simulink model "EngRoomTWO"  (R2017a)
settings: Solver=VariableStepAuto  StartTime=0.0  StopTime=10.0  RelTol=1e-3
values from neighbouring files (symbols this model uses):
  EngDat = engine_pre()    [run_master.m]    (also in engine_pre.m = [MCR1, BSFC1, x)
undefined symbols (not defined in the file or in its folder): num

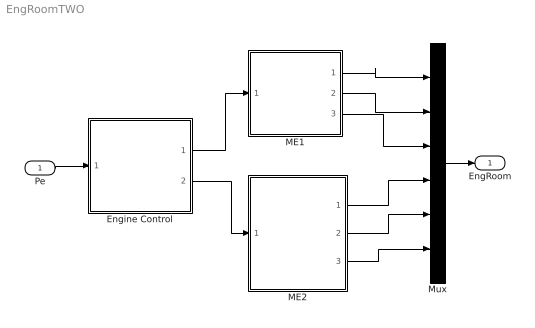
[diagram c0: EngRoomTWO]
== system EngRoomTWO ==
  Pe : Inport
  Engine Control : MATLAB Function  TreatAsAtomicUnit=on
  ME1 : MATLAB Function  TreatAsAtomicUnit=on
  ME2 : MATLAB Function  TreatAsAtomicUnit=on
  Mux : Mux  Inputs=6
  EngRoom : Outport
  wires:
  Pe/1 -> Engine Control/1(Pe)
  Engine Control/1(P1) -> ME1/1("Pb ")
  Engine Control/2(P2) -> ME2/1("Pb ")
  ME1/3(x) -> Mux/3
  ME2/3(x) -> Mux/6
  ME2/2(Pb) -> Mux/5
  ME2/1(fuel_cons) -> Mux/4
  ME1/2(Pb) -> Mux/2
  ME1/1(fuel_cons) -> Mux/1
  Mux/1 -> EngRoom/1

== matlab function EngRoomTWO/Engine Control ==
function [P1, P2] = fcn(Pe,EngDat)
%take in the total propulsive powering need
%find the optimal settings so that each engine runs close to optimum
%output the load (and rpm) for each engine

%Pe is the required effective power to overcome resistance, the break power
%needed from the engineroom depends on the efficiency of the propulsion
%system, which in turn depends on the configuration of the engines and
%propulsors
% PMCR1=0;
% PMCR2=0;
% load=0;
%capacity of each engine
PMCR1=EngDat(1,1);
PMCR2=EngDat(2,1);

% x=EngDat(1,3);

%pre-set to 0
P1=0;
P2=0;

%% Convert Pe into Pb required from the machinery
eta_D = 0.55;
eta_M = 0.95*0.98;
eta_T = eta_D* eta_M;   %Total efficiency
Pb = (Pe/eta_T); %kW

%%Find the required loading for the engines     
        if Pb<=PMCR2 % If the required load is less than capacity of eng 2
            P1=0; 
            P2=Pb;
            return
        elseif Pb<=PMCR1 % If the required load is less than capacity of eng 2
            P2=0;
            P1=Pb;
            return
        else
            load=Pb/(PMCR1+PMCR2);
            P1=load*PMCR1;
            P2=load*PMCR2;
            
        end
    
end

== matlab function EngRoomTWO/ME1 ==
function [fuel_cons, Pb, x] = fcn(Pb, num, EngDat)


PMCR=EngDat(1,1);
x = Pb/PMCR; %percentage of maximum
BSFC=EngDat(1,2); %g/kWh
delta_BSFC = 0;% 6610.6*x^6 - 20524*x^5 + 23791*x^4 - 11985*x^3 + 1803.2*x^2 + 340.12*x - 36.733;


fuel_cons = ((delta_BSFC+BSFC)*Pb)/(1000*4); %kg/15 min


end

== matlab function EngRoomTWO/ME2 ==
function [fuel_cons, Pb, x] = fcn(Pb, num, EngDat)


PMCR=EngDat(2,1);
x = Pb/PMCR; %percentage of maximum
BSFC=EngDat(2,2); %g/kWh
delta_BSFC = 0;%6610.6*x^6 - 20524*x^5 + 23791*x^4 - 11985*x^3 + 1803.2*x^2 + 340.12*x - 36.733;


fuel_cons = ((delta_BSFC+BSFC)*Pb)/(1000*4); %kg/15min


end
